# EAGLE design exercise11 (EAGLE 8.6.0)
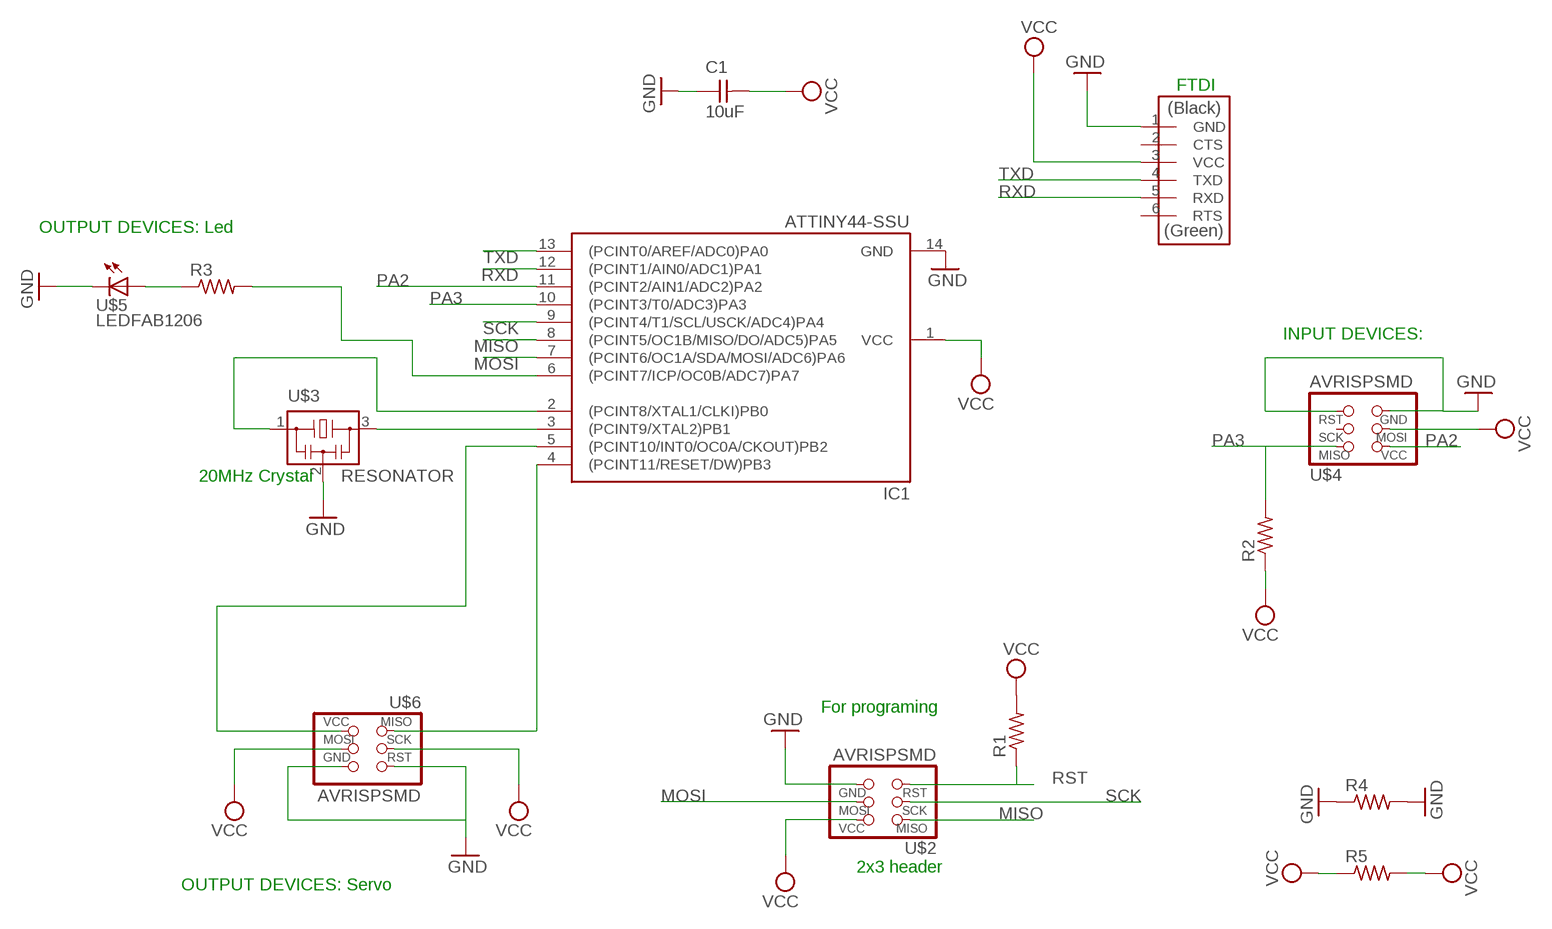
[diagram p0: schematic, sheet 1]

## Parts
C1  10uF  CAP-UNPOLARIZEDFAB  [C1206FAB]
IC1  ATTINY44-SSU  [SOIC14]
R1  RES-US1206FAB  [R1206FAB]
R2  RES-US1206FAB  [R1206FAB]
R3  RES-US1206FAB  [R1206FAB]
R4  RES-US1206FAB  [R1206FAB]
R5  RES-US1206FAB  [R1206FAB]
U$1  FTDI-SMD-HEADER  [1X06SMD]
U$2  AVRISPSMD  [2X03SMD]
U$3  RESONATOR  [EFOBM]
U$4  AVRISPSMD  [2X03SMD]
U$5  LEDFAB1206  [LED1206FAB]
U$6  AVRISPSMD  [2X03SMD]

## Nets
GND: C1.1 IC1.14(GND) R4.1 R4.2 U$1.1(GND) U$2.6(GND) U$3.2 U$4.5(RST) U$4.6(GND) U$5.2(C) U$6.5(RST) U$6.6(GND)
MISO: IC1.8((PCINT5/OC1B/MISO/DO/ADC5)PA5) U$2.1(MISO)
MOSI: IC1.7((PCINT6/OC1A/SDA/MOSI/ADC6)PA6) U$2.4(MOSI)
N$1: IC1.2((PCINT8/XTAL1/CLKI)PB0) U$3.1
N$2: IC1.3((PCINT9/XTAL2)PB1) U$3.3
N$3: R3.1 U$5.1(A)
N$4: IC1.6((PCINT7/ICP/OC0B/ADC7)PA7) R3.2
N$5: IC1.5((PCINT10/INT0/OC0A/CKOUT)PB2) U$6.2(VCC)
N$7: IC1.4((PCINT11/RESET/DW)PB3) U$6.1(MISO)
PA2: IC1.11((PCINT2/AIN1/ADC2)PA2) U$4.2(VCC)
PA3: IC1.10((PCINT3/T0/ADC3)PA3) R2.2 U$4.1(MISO)
RST: R1.1 U$2.5(RST)
RXD: IC1.12((PCINT1/AIN0/ADC1)PA1) U$1.5(RXD)
SCK: IC1.9((PCINT4/T1/SCL/USCK/ADC4)PA4) U$2.3(SCK)
TXD: IC1.13((PCINT0/AREF/ADC0)PA0) U$1.4(TXD)
VCC: C1.2 IC1.1(VCC) R1.2 R2.1 R5.1 R5.2 U$1.3(VCC) U$2.2(VCC) U$4.4(MOSI) U$6.3(SCK) U$6.4(MOSI)
Unconnected: U$1.2(CTS) U$1.6(RTS) U$4.3(SCK)

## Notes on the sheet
- FTDI
- OUTPUT DEVICES: Led
- INPUT DEVICES:
- 20MHz Crystal
- For programing
- 2x3 header
- OUTPUT DEVICES: Servo

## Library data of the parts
C1 = fab:CAP-UNPOLARIZED
IC1 = fab:ATTINY44
R1-R5 = fab:RES-US: Resistor (US Symbol)
U$1 = fab:FTDI-SMD-HEADER
U$2 U$4 U$6 = fab:AVRISP
U$3 = fab:RESONATOR
U$5 = fab:LED: LED

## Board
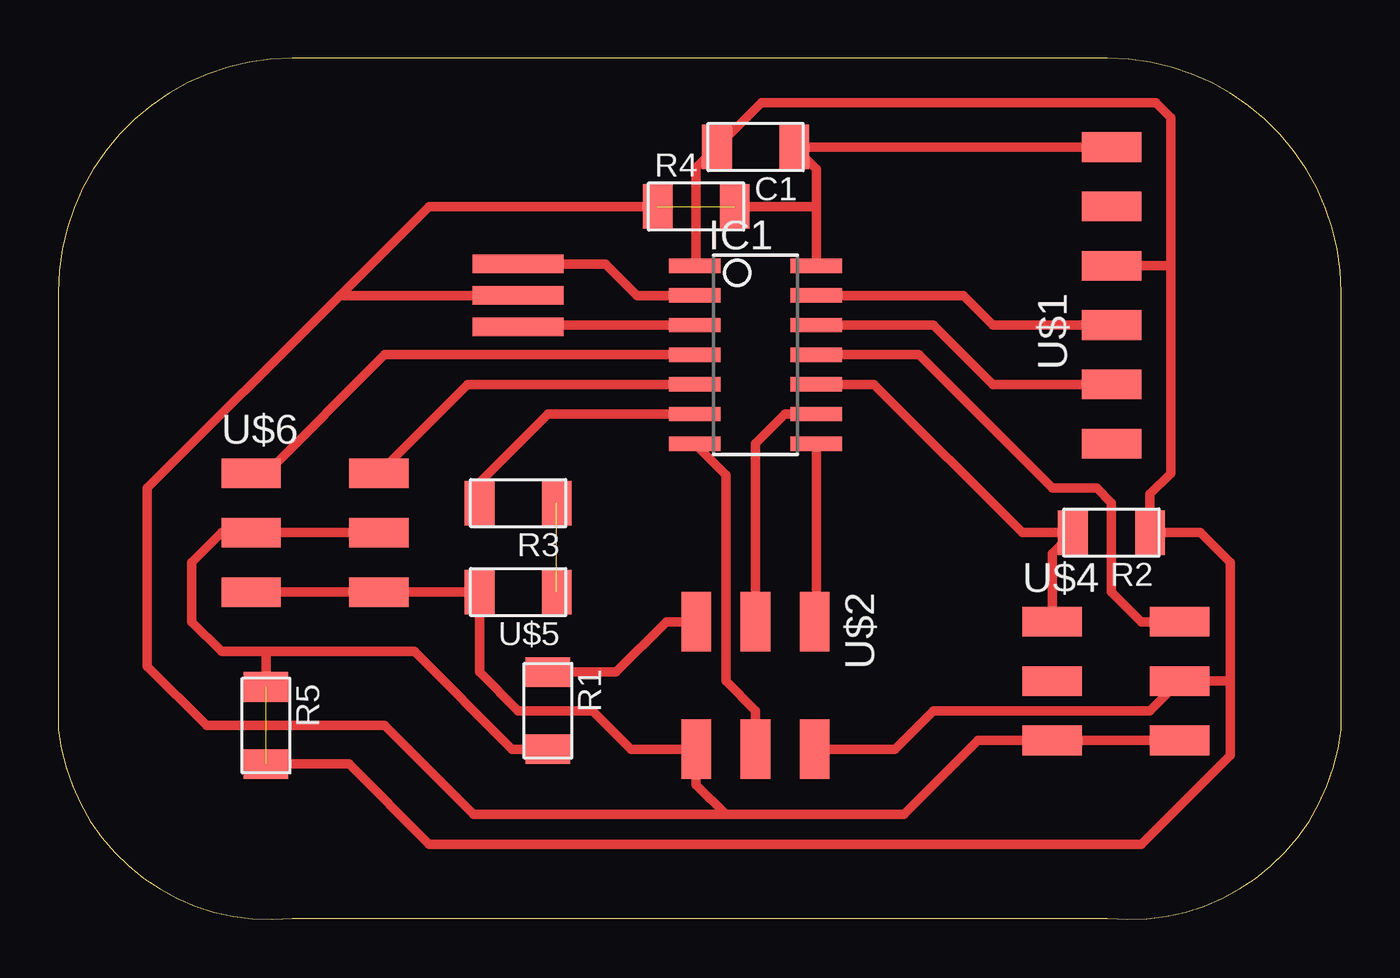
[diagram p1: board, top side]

Size 54.91 x 36.87 mm. Coordinates in mm from the lower left corner, seen from the top.
Outline: 0,26.87 0,8.14 arc90 10,0.05 44.91,0.05 arc90 54.91,8.14 54.91,26.87 arc90 44.91,36.87 10,36.87 arc90 0,26.87
Copper layers (1*16): Top 0.035mm / dielectric 1.5mm / Bottom 0.035mm
Design rules "default": minimum track width 6mil, minimum drill 0.35mm, track to track 6mil, track to pad 6mil, pad to pad 6mil, via to via 6mil, smd to smd 6mil, copper to edge 40mil, drill to drill 6mil, minimum pad ring 10mil, minimum via ring 8mil, stop-mask expansion 4mil, vias tented up to drill 0mil, thermal gap 10mil

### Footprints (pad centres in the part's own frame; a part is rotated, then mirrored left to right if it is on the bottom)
C1206FAB = smd 1.27 x 1.905: 1 -1.651,0; 2 1.651,0
SOIC14 = smd 0.61 x 2.21: 1 -3.81,-2.603; 2 -2.54,-2.603; 3 -1.27,-2.603; 4 0,-2.603; 5 1.27,-2.603; 6 2.54,-2.603; 7 3.81,-2.603; 8 3.81,2.603; 9 2.54,2.603; 10 1.27,2.603; 11 0,2.603; 12 -1.27,2.603; 13 -2.54,2.603; 14 -3.81,2.603
R1206FAB = smd 1.27 x 1.905: 1 -1.651,0; 2 1.651,0
1X06SMD = smd 2.54 x 1.27: 1 0,6.35; 2 0,3.81; 3 0,1.27; 4 0,-1.27; 5 0,-3.81; 6 0,-6.35
2X03SMD = smd 2.54 x 1.27: 1 -2.54,2.54; 2 2.92,2.54; 3 -2.54,0; 4 2.92,0; 5 -2.54,-2.54; 6 2.92,-2.54
EFOBM = smd 0.8 x 3.9: 1 -1.35,0; 2 0,0; 3 1.35,0
LED1206FAB = smd 1.27 x 1.905: 1 -1.651,0; 2 1.651,0

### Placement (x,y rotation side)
C1  29.85,33.07 180 top
IC1  29.85,24.18 270 top
R1  20.96,8.94 270 top
R2  45.08,16.56 180 top
R3  19.68,17.83 180 top
R4  27.3,30.53 0 top
R5  8.89,8.3 270 top
U$1  45.08,26.72 0 top
U$2  29.85,10.21 270 top
U$3  19.68,26.72 270 top
U$4  45.08,10.21 0 top
U$5  19.68,14.02 180 top
U$6  10.79,16.56 0 top

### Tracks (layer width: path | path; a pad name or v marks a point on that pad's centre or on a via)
GND  (1 unrouted)
  Top 0.406: U$1.1 C1.1 32.45,32.12 32.45,30.53 | IC1.14 32.45,30.53 | U$4.6 U$4.5 39.37,7.67 36.19,4.49 28.57,4.49 | U$6.5 U$6.6 U$5.2 18.03,10.59 19.68,8.94 22.86,8.94 24.51,7.29 U$2.6 27.3,5.76 28.57,4.49 | 12.07,26.72 3.81,18.46 3.81,10.84 6.35,8.3 13.97,8.3 17.78,4.49 28.57,4.49 | U$3.2 12.07,26.72 | 12.07,26.72 15.87,30.53 R4.1 | R4.2 32.45,30.53
MISO
  Top 0.406: U$2.1 32.45,12.81 IC1.8
MOSI
  Top 0.406: U$2.4 29.85,8.94 28.57,10.21 28.57,19.04 IC1.7
N$1
  Top 0.406: 27.22,26.8 27.3,26.72 IC1.2 24.76,26.72 23.41,28.07 U$3.1
N$2
  Top 0.406: U$3.3 19.76,25.45 IC1.3
N$3  (1 unrouted)
N$4
  Top 0.406: R3.2 18.03,18.72 20.96,21.64 IC1.6
N$5
  Top 0.406: 13.71,19.48 U$6.2 17.53,22.91 IC1.5
N$7
  Top 0.406: U$6.1 8.89,19.1 13.97,24.18 IC1.4
PA2
  Top 0.406: U$4.2 46.35,12.75 45.08,14.02 45.08,17.83 44.45,18.46 42.55,18.46 36.83,24.18 IC1.11
PA3
  Top 0.406: IC1.10 34.92,22.91 41.27,16.56 R2.2 42.55,15.67 U$4.1
RST
  Top 0.406: R1.1 23.88,10.59 26.04,12.75 U$2.5
RXD
  Top 0.406: IC1.12 37.47,25.45 40,22.91 U$1.5
SCK
  Top 0.406: U$2.3 29.85,20.37 31.11,21.64 IC1.9
TXD
  Top 0.406: IC1.13 38.73,26.72 40,25.45 U$1.4
VCC  (1 unrouted)
  Top 0.406: IC1.1 27.3,28.05 27.3,32.18 C1.2 30.1,34.97 46.99,34.97 47.62,34.34 47.62,27.99 | U$1.3 47.62,27.99 | 47.62,27.99 47.62,19.1 46.74,18.21 R2.1 48.89,16.56 50.16,15.29 50.16,10.21 | 50.16,10.21 U$4.4 46.73,8.94 37.47,8.94 35.81,7.29 U$2.2 | U$6.4 U$6.3 6.98,16.56 5.71,15.29 5.71,12.75 6.98,11.48 8.89,11.48 | R1.2 19.43,7.29 15.24,11.48 8.89,11.48 | R5.1 8.89,11.48 | 50.16,10.21 50.16,7.03 46.35,3.22 15.87,3.22 12.45,6.65 R5.2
